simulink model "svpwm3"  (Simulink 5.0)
settings: Solver=ode45  StartTime=0  StopTime=.02  MaxStep=1e-6  RelTol=1e-3
InitFcn:
  | warning off;clc;fout=50;fsw=20000;disp(' Output frequency Switching frequency  [Hz] :  ');
  | disp('         fout       fsw');disp([fout   fsw])
libraries: simulink x2, simulink_extras x1

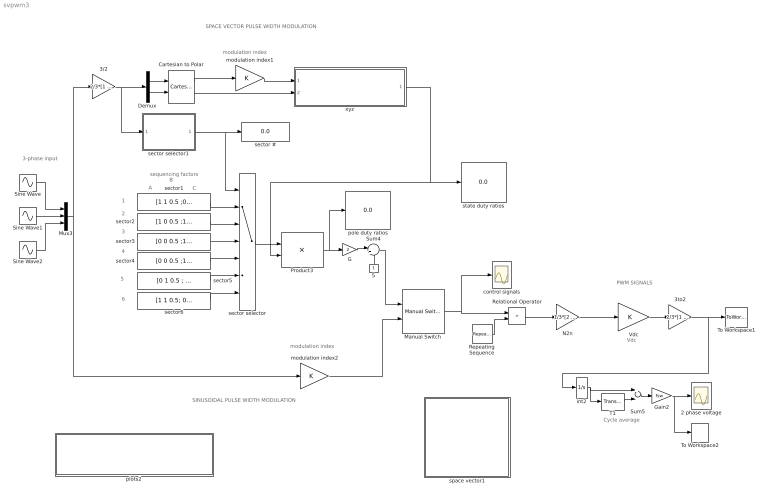
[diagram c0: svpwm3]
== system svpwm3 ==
  note: SPACE VECTOR PULSE WIDTH MODULATION
  note: sequencing factors
  note: 1
  note: 2
  note: 3
  note: 4
  note: 5
  note: 6
  note: A
  note: B
  note: C
  note: modulation index
  note: PWM SIGNALS
  note: Cycle average
  note: SINUSOIDAL PULSE WIDTH MODULATION
  note: modulation index
  note: 3-phase input
  note: Vdc
  2 phase voltage : Scope
  3/2 : Gain  Gain=2/3*[1 -0.5 -0.5;0 sqrt(3)/2 -sqrt(3)/2]  Multiplication=Matrix(K*u)
  3to2 : Gain  Gain=2/3*[1 -0.5 -0.5;0 sqrt(3)/2 -sqrt(3)/2]  Multiplication=Matrix(K*u)
  5 : Constant  Orientation=up
  Cartesian to Polar : simulink_extras/Transformations/Cartesian to Polar
  Demux : Demux  Outputs=2
  G : Gain  Gain=2
  Gain2 : Gain  Gain=fsw
  Manual Switch : simulink/Signal Routing/Manual Switch  sw=1  action=0
  Mux3 : Mux  Inputs=3
  N2n : Gain  Gain=1/3*[2 -1 -1;-1 2 -1;-1 -1 2]  Multiplication=Matrix(K*u)
  Product3 : Product  Multiplication=Matrix(*)
  Relational Operator : RelationalOperator  Operator=>
  Repeating Sequence : simulink/Sources/Repeating Sequence  rep_seq_t="[0  0.5/fsw 1/fsw]"  rep_seq_y=[1 -1 1]
  Sine Wave : Sin  Frequency=2*pi*fout  Phase=pi/2  SampleTime=0
  Sine Wave1 : Sin  Frequency=2*pi*fout  Phase=pi/2 -2*pi/3  SampleTime=0
  Sine Wave2 : Sin  Frequency=2*pi*fout  Phase=pi/2+2*pi/3  SampleTime=0
  Sum4 : Sum  Inputs=|+-
  Sum5 : Sum  Inputs=+-
  T1 : TransportDelay  DelayTime=1/fsw
  To Workspace1 : ToWorkspace  VariableName=abpwm  SampleTime=-1  SaveFormat=Array
  To Workspace2 : ToWorkspace  VariableName=ab  SampleTime=-1  SaveFormat=Array
  Vdc : Gain
  control signals : Scope
  int2 : Integrator
  modulation index1 : Gain
  modulation index2 : Gain
  plots2 : Subsystem
  pole duty ratios : Display
  sector selector : MultiPortSwitch  Inputs=6
  sector # : Display
  sector selector1 : Subsystem
  sector1 : Constant  Value=[1 1 0.5 ;0 1 0.5;0 0 0.5]
  sector2 : Constant  Value=[1 0 0.5 ;1 1 0.5; 0 0 0.5]  VectorParams1D=off
  sector3 : Constant  Value=[0 0 0.5 ;1 1 0.5; 0 1 0.5]  VectorParams1D=off
  sector4 : Constant  Value=[0 0 0.5 ;1 0 0.5; 1 1 0.5]
  sector5 : Constant  Value=[0 1 0.5 ; 0 0 0.5; 1 1 0.5]  VectorParams1D=off
  sector6 : Constant  Value=[1 1 0.5; 0 0 0.5; 1 0 0.5]  VectorParams1D=off
  space vector1 : Subsystem
  state duty ratios : Display
  xyz : Subsystem
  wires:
  sector2/1 -> sector selector/3
  sector1/1 -> sector selector/2
  sector3/1 -> sector selector/4
  5/1 -> Sum4/2
  G/1 -> Sum4/1
  Demux/2 -> Cartesian to Polar/2
  Demux/1 -> Cartesian to Polar/1
  Cartesian to Polar/1 -> modulation index1/1
  sector4/1 -> sector selector/5
  sector5/1 -> sector selector/6
  sector6/1 -> sector selector/7
  sector selector1/1(sector) -> sector selector/1, sector #/1
  sector selector/1 -> Product3/1
  Product3/1 -> G/1, pole duty ratios/1
  xyz/1(xyz) -> Product3/2, state duty ratios/1
  Repeating Sequence/1 -> Relational Operator/2
  T1/1 -> Sum5/2
  int2/1 -> Sum5/1, T1/1
  Sum5/1 -> Gain2/1
  Gain2/1 -> 2 phase voltage/1, To Workspace2/1
  Sine Wave/1 -> Mux3/1
  Sine Wave1/1 -> Mux3/2
  Sine Wave2/1 -> Mux3/3
  Sum4/1 -> Manual Switch/1
  Manual Switch/1 -> Relational Operator/1, control signals/1
  modulation index2/1 -> Manual Switch/2
  Mux3/1 -> modulation index2/1, 3/2/1
  3/2/1 -> Demux/1, sector selector1/1(fs)
  3to2/1 -> To Workspace1/1, int2/1
  Vdc/1 -> 3to2/1
  Relational Operator/1 -> N2n/1
  N2n/1 -> Vdc/1
  modulation index1/1 -> xyz/1(amp)
  Cartesian to Polar/2 -> xyz/2(phase)

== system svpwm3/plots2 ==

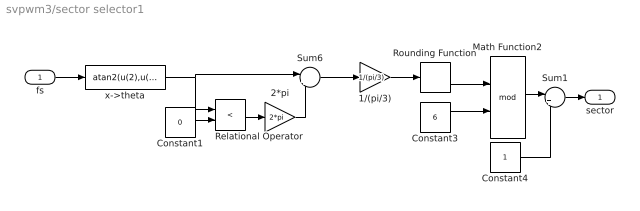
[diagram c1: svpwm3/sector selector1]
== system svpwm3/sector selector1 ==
  fs : Inport
  1/(pi/3) : Gain  Gain=1/(pi/3)
  2*pi : Gain  Gain=2*pi
  Constant1 : Constant  Value=0
  Constant3 : Constant  Value=6
  Constant4 : Constant
  Math Function2 : Math  Operator=mod
  Relational Operator : RelationalOperator  Operator=<
  Rounding Function : Rounding
  Sum1 : Sum  Inputs=|++
  Sum6 : Sum  Inputs=|++
  x->theta : Fcn  Expr=atan2(u(2),u(1))
  sector : Outport
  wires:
  Constant1/1 -> Relational Operator/2
  Relational Operator/1 -> 2*pi/1
  2*pi/1 -> Sum6/2
  1/(pi/3)/1 -> Rounding Function/1
  Rounding Function/1 -> Math Function2/1
  Constant3/1 -> Math Function2/2
  fs/1 -> x->theta/1
  x->theta/1 -> Relational Operator/1, Sum6/1
  Sum1/1 -> sector/1
  Math Function2/1 -> Sum1/1
  Constant4/1 -> Sum1/2
  Sum6/1 -> 1/(pi/3)/1

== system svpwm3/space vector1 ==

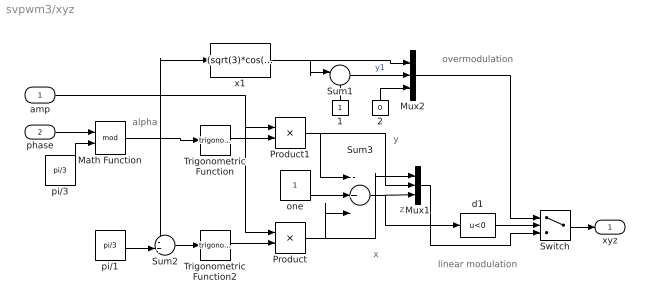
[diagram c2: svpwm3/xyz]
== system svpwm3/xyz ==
  note: alpha
  note: y
  note: x
  note: z
  note: overmodulation
  note: linear modulation
  amp : Inport
  phase : Inport  Port=2
  1 : Constant  Orientation=up
  2 : Constant  Orientation=up  Value=0
  Math Function : Math  Operator=mod
  Mux1 : Mux  Inputs=3
  Mux2 : Mux  Inputs=3
  Product : Product
  Product1 : Product
  Sum1 : Sum  Inputs=|-+
  Sum2 : Sum  Inputs=-+|
  Sum3 : Sum  Inputs=-+-|
  Switch : Switch  Threshold=0.5
  Trigonometric Function : Trigonometry
  Trigonometric Function2 : Trigonometry
  d1 : Fcn  Expr=u<0
  one : Constant
  pi/1 : Constant  Value=pi/3
  pi/3 : Constant  Value=pi/3
  x1 : Fcn  Expr=(sqrt(3)*cos(u)-sin(u))/(sqrt(3)*cos(u)+sin(u))
  xyz : Outport
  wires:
  pi/1/1 -> Sum2/2
  Math Function/1 -> Trigonometric Function/1, Sum2/1, x1/1
  Sum2/1 -> Trigonometric Function2/1
  Trigonometric Function/1 -> Product1/2
  Trigonometric Function2/1 -> Product/2
  amp/1 -> Product/1, Product1/1
  pi/3/1 -> Math Function/2
  Product1/1 -> Mux1/2, Sum3/1
  Product/1 -> Mux1/1, Sum3/3
  one/1 -> Sum3/2
  Sum3/1 -> Mux1/3, d1/1
  d1/1 -> Switch/2
  x1/1 -> Mux2/1, Sum1/1
  Sum1/1 -> Mux2/2  "y1"
  2/1 -> Mux2/3
  1/1 -> Sum1/2
  Mux1/1 -> Switch/3
  Mux2/1 -> Switch/1
  phase/1 -> Math Function/1
  Switch/1 -> xyz/1
